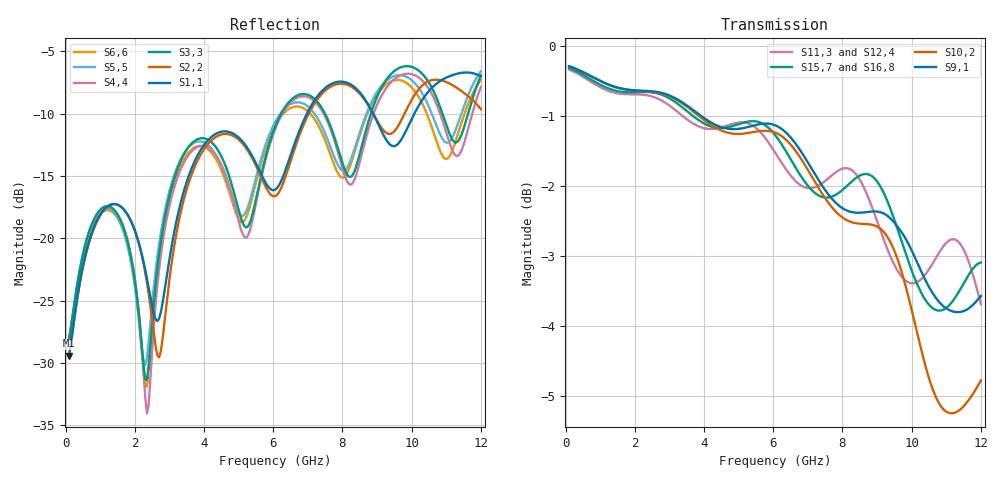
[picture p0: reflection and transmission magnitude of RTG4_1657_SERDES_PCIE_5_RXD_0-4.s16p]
! RTG4 1657 S-parameter file
! Microsemi Corporation (c) 2019
!Initial ver: Jul 30, 2019
! Port::PIN_NAME::NET_NAME::S-parameter ports::PORT SIDE
! Port1:--:SERDES_PCIE_5_RXD0_N_DIE::1::DIE
! Port2:--:SERDES_PCIE_5_RXD0_P_DIE::2::DIE
! Port3:AY33:SERDES_PCIE_5_RXD0_N_BGA::3::BGA
! Port4:BA33:SERDES_PCIE_5_RXD0_P_BGA::4::BGA
! Port5:--:SERDES_PCIE_5_RXD1_N_DIE::5::DIE
! Port6:--:SERDES_PCIE_5_RXD1_P_DIE::6::DIE
! Port7:AY35:SERDES_PCIE_5_RXD1_N_BGA::7::BGA
! Port8:BA35:SERDES_PCIE_5_RXD1_P_BGA::8::BGA
! Port9:--:SERDES_PCIE_5_RXD2_N_DIE::9::DIE
! Port10:--:SERDES_PCIE_5_RXD2_P_DIE::10::DIE
! Port11:AY37:SERDES_PCIE_5_RXD2_N_BGA::11::BGA
! Port12:BA37:SERDES_PCIE_5_RXD2_P_BGA::12::BGA
! Port13:--:SERDES_PCIE_5_RXD3_N_DIE::13::DIE
! Port14:--:SERDES_PCIE_5_RXD3_P_DIE::14::DIE
! Port15:AV38:SERDES_PCIE_5_RXD3_N_BGA::15::BGA
! Port16:AW38:SERDES_PCIE_5_RXD3_P_BGA::16::BGA
!TouchstoneFormatFlag = 1
! GNDNET
! NETSLIST
! User Comments:
! Touchstone file exported from HFSS 2018.2.0
!  File:  //LSI_Z840_SIM_PC/Simulation_Data/MASUMISU/Microsemi_190710/YBD197_150320_NETCHANGE_SERDES_PCIE_5_RXD.aedt
!  Generated:  9:22:14 ??  7 16, 2019
!  Design:  HFSSModel1
!  Project:  YBD197_150320_NETCHANGE_SERDES_PCIE_5_RXD
!  Setup:  Setup1
!  Solution:  Sweep
! Terminal data exported
! Port[1] = SERDES_PCIE_5_RXD0_N_DIE
! Port[2] = SERDES_PCIE_5_RXD0_P_DIE
! Port[3] = SERDES_PCIE_5_RXD1_N_DIE
! Port[4] = SERDES_PCIE_5_RXD1_P_DIE
! Port[5] = SERDES_PCIE_5_RXD2_N_DIE
! Port[6] = SERDES_PCIE_5_RXD2_P_DIE
! Port[7] = SERDES_PCIE_5_RXD3_N_DIE
! Port[8] = SERDES_PCIE_5_RXD3_P_DIE
! Port[9] = SERDES_PCIE_5_RXD0_N_BGA
! Port[10] = SERDES_PCIE_5_RXD0_P_BGA
! Port[11] = SERDES_PCIE_5_RXD1_N_BGA
! Port[12] = SERDES_PCIE_5_RXD1_P_BGA
! Port[13] = SERDES_PCIE_5_RXD2_N_BGA
! Port[14] = SERDES_PCIE_5_RXD2_P_BGA
! Port[15] = SERDES_PCIE_5_RXD3_N_BGA
! Port[16] = SERDES_PCIE_5_RXD3_P_BGA
# GHZ S DB R 50.000000
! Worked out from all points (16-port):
!   239 points, 100 MHz to 12 GHz, reference 50 ohm
!   strongest paths, dB at 100 MHz, 3.05 GHz, 6.05 GHz, 9.05 GHz, 12 GHz:
!     S9,1: -0.3, -0.7, -1.1, -2.4, -3.6
!     S10,2: -0.3, -0.7, -1.2, -2.6, -4.8
!     S15,7: -0.3, -0.8, -1.3, -2.0, -3.1
!     S16,8: -0.3, -0.7, -1.3, -1.9, -3.1
!     S11,3: -0.3, -0.9, -1.5, -2.6, -3.7
!     S12,4: -0.3, -0.9, -1.6, -2.9, -3.8
!   lowest |S11| = -29.4 dB at 100 MHz (marker M1), VSWR 1.07, Z = 53 - j1.81 ohm
!   |S11| at or under -10 dB: start of sweep to 6.973 GHz; 8.885 GHz to 10.08 GHz (1.193 GHz wide, 12.6 % of centre)
